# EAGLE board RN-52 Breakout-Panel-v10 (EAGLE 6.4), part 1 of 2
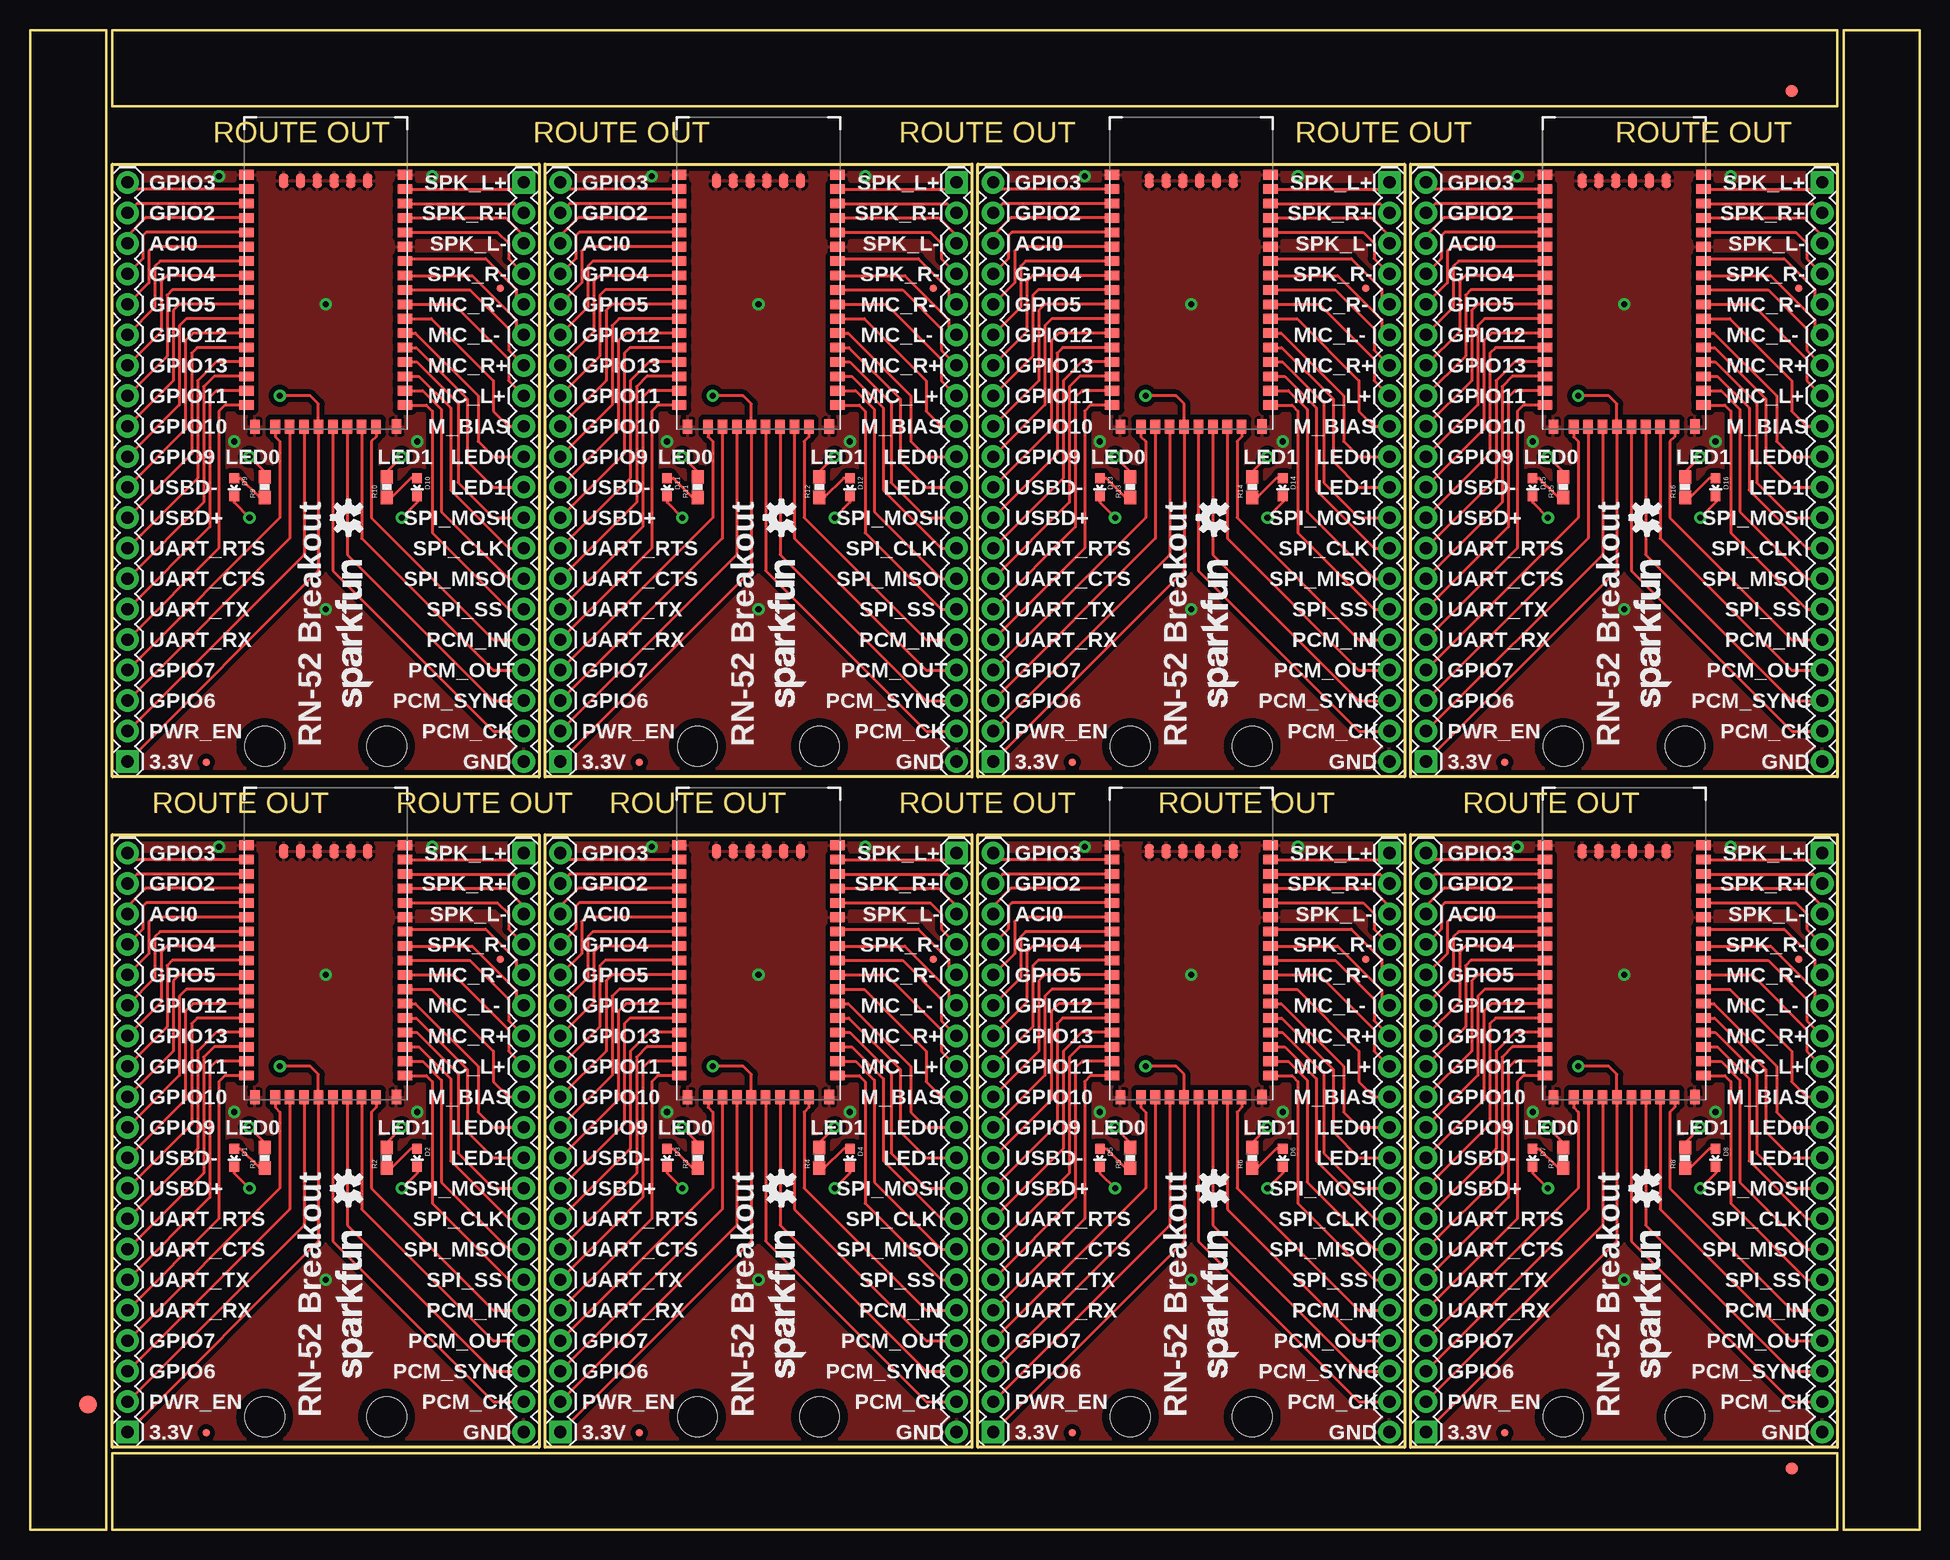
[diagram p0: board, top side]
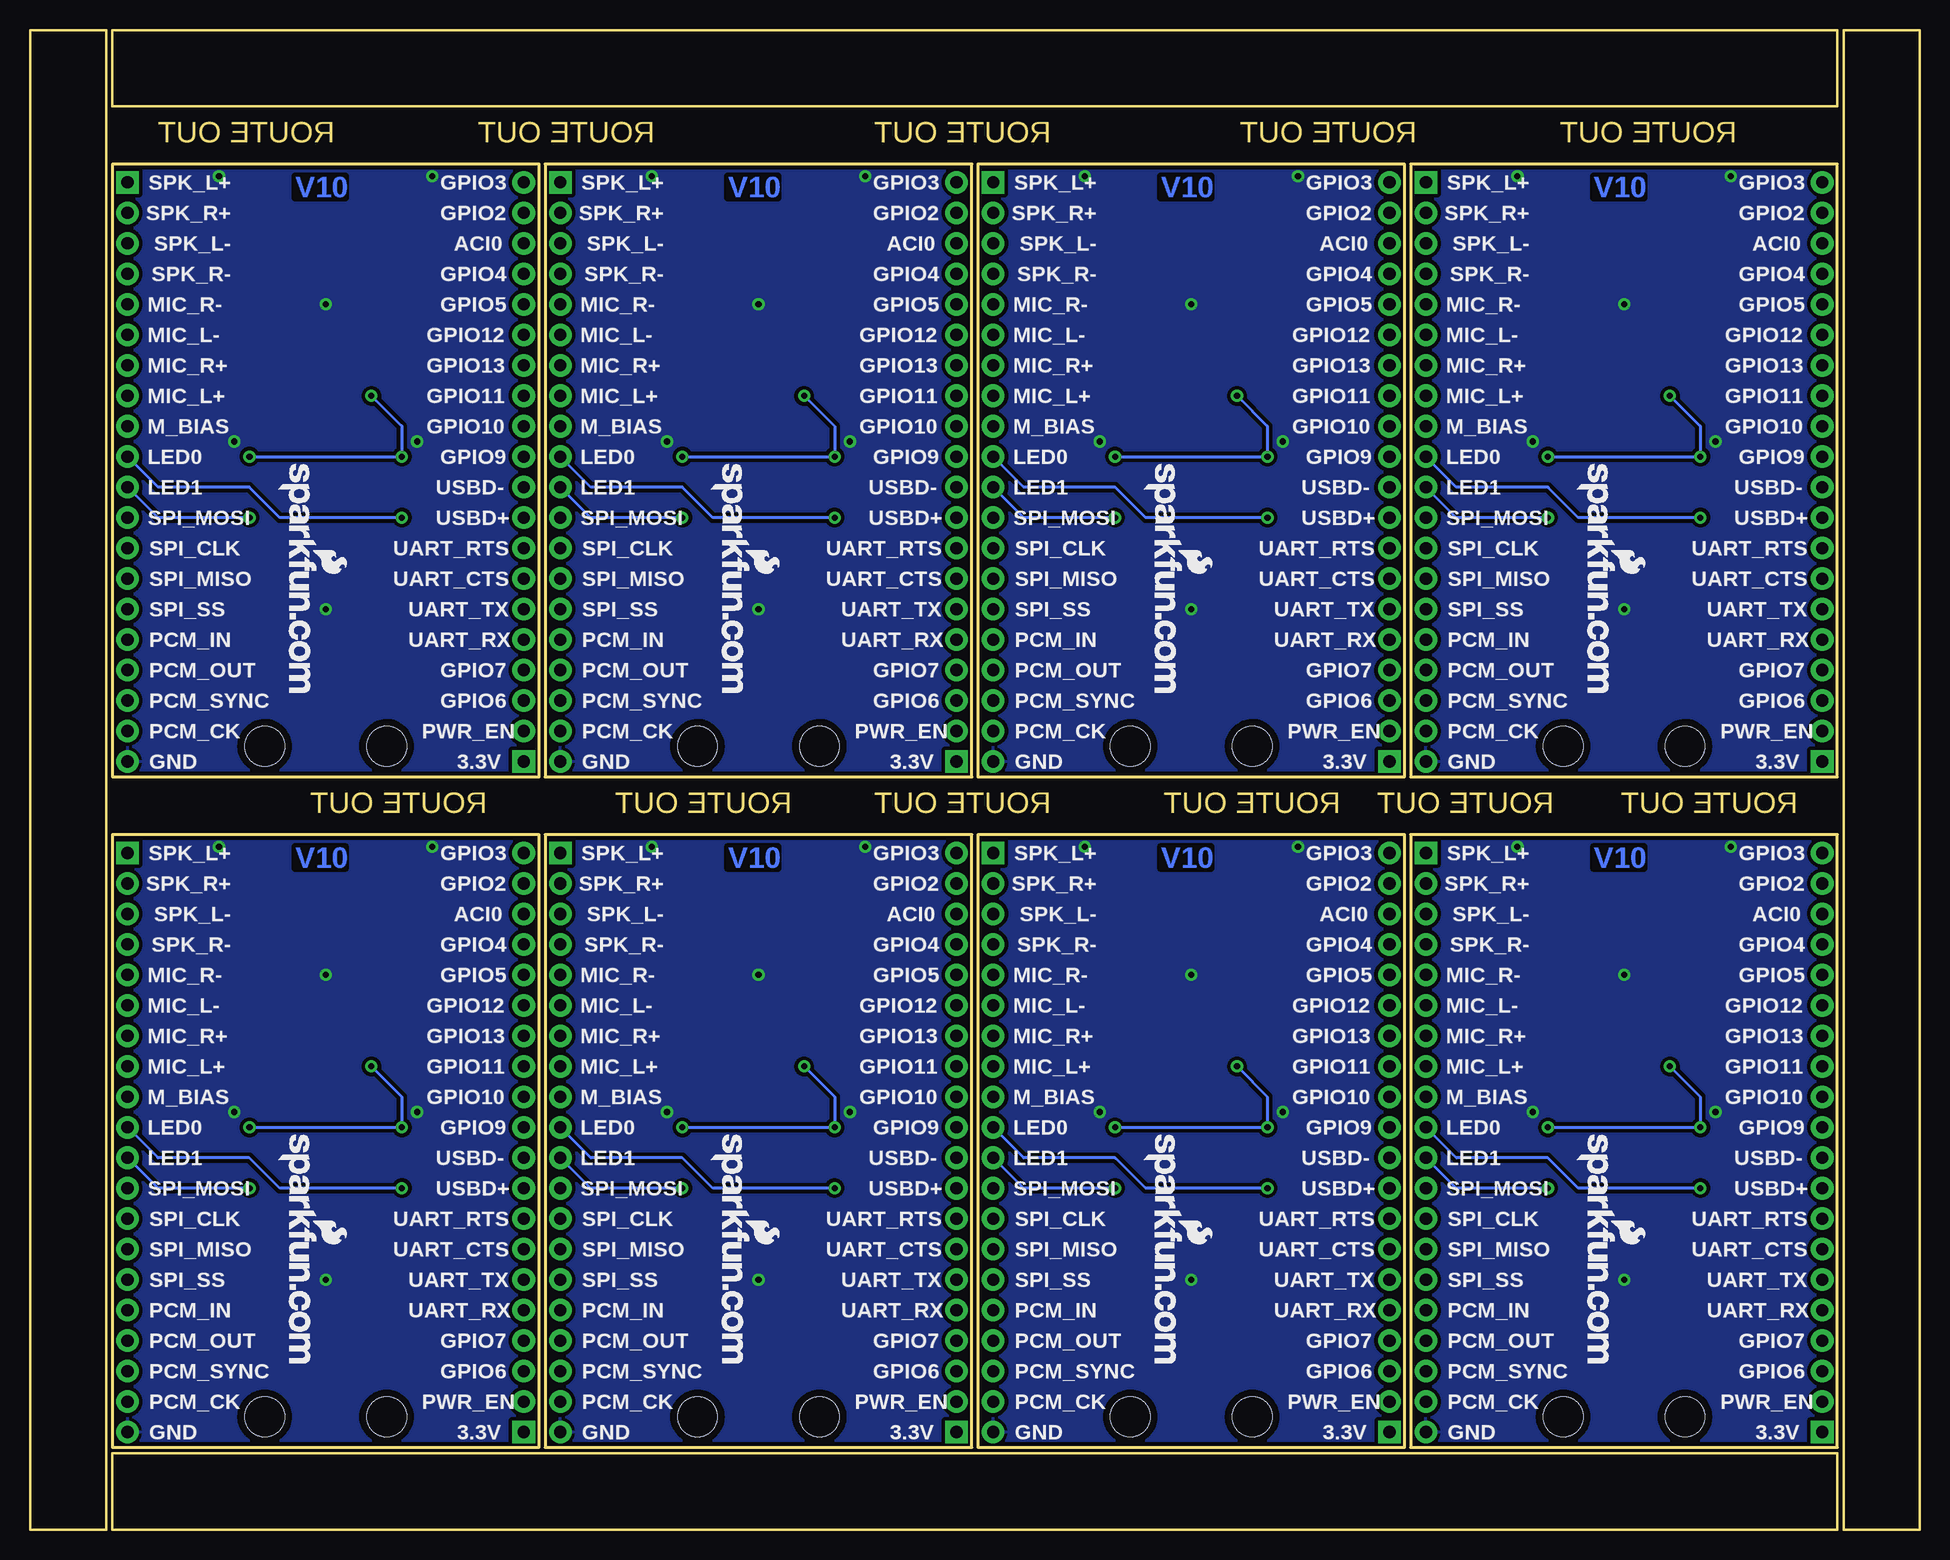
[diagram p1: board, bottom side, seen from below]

Size 157.48 x 124.97 mm. Coordinates in mm from the lower left corner, seen from the top.
Outline: 6.86,57.91 42.42,57.91 42.42,6.86 6.86,6.86 6.86,57.91
Outline: 42.93,57.91 78.49,57.91 78.49,6.86 42.93,6.86 42.93,57.91
Outline: 78.99,57.91 114.55,57.91 114.55,6.86 78.99,6.86 78.99,57.91
Outline: 115.06,57.91 150.62,57.91 150.62,6.86 115.06,6.86 115.06,57.91
Outline: 6.86,113.79 42.42,113.79 42.42,62.74 6.86,62.74 6.86,113.79
Outline: 42.93,113.79 78.49,113.79 78.49,62.74 42.93,62.74 42.93,113.79
Outline: 78.99,113.79 114.55,113.79 114.55,62.74 78.99,62.74 78.99,113.79
Outline: 115.06,113.79 150.62,113.79 150.62,62.74 115.06,62.74 115.06,113.79
Outline: 6.35,0 6.35,124.97 0,124.97 0,0 6.35,0
Outline: 6.86,0 150.62,0 150.62,6.35 6.86,6.35 6.86,0
Outline: 157.48,0 157.48,124.97 151.13,124.97 151.13,0 157.48,0
Outline: 6.86,118.62 150.62,118.62 150.62,124.97 6.86,124.97 6.86,118.62
Copper layers (1*16): Top 0.035mm / dielectric 1.5mm / Bottom 0.035mm
Design rules "default *": minimum track width 7mil, minimum drill 15mil, track to track 8mil, track to pad 8mil, pad to pad 8mil, via to via 8mil, smd to smd 8mil, copper to edge 8mil, drill to drill 8mil, minimum pad ring 12mil, minimum via ring 10mil, stop-mask expansion 4mil, vias tented up to drill 20mil, thermal gap 10mil

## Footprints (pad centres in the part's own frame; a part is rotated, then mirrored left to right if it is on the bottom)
LED-0603 = smd 0.8 x 0.8: A 0,-0.75; C 0,0.75
MICRO-FIDUCIAL = smd 0.635 x 0.635: 1 0,0
FIDUCIAL-1.5X3 = smd 1.5 x 1.5: 1 0,0
FIDUCIAL-1X2 = smd 1 x 1: 1 0,0
1X20 = drill 1.016 pad 1.88 square: 1 0,0 | drill 1.016 pad 1.88: 2 2.54,0; 3 5.08,0; 4 7.62,0; 5 10.16,0; 6 12.7,0; 7 15.24,0; 8 17.78,0; 9 20.32,0; 10 22.86,0; 11 25.4,0; 12 27.94,0; 13 30.48,0; 14 33.02,0; 15 35.56,0; 16 38.1,0; 17 40.64,0; 18 43.18,0; 19 45.72,0; 20 48.26,0
0603-RES = smd 1.1 x 1: 1 -0.85,0; 2 0.85,0
STAND-OFF = hole 3.302: 0,0
RN-52 = smd 1.2 x 0.8: 1 -6.6,8.33; 2 -6.6,7.13; 3 -6.6,5.93; 4 -6.6,4.73; 5 -6.6,3.53; 6 -6.6,2.33; 7 -6.6,1.13; 8 -6.6,-0.07; 9 -6.6,-1.27; 10 -6.6,-2.47; 11 -6.6,-3.67; 12 -6.6,-4.87; 13 -6.6,-6.07; 14 -6.6,-7.27; 15 -6.6,-8.47; 16 -6.6,-9.67; 25 6.6,-9.67; 26 6.6,-8.47; 27 6.6,-7.27; 28 6.6,-6.07; 29 6.6,-4.87; 30 6.6,-3.67; 31 6.6,-2.47; 32 6.6,-1.27; 33 6.6,-0.07; 34 6.6,1.13; 35 6.6,2.33; 36 6.6,3.53; 37 6.6,4.73; 38 6.6,5.93; 39 6.6,7.13; 40 6.6,8.33; G1 -6.6,9.53; G4 6.6,9.53 | smd 0.8 x 1.2: 17 -4.2,-11.47; 18 -3,-11.47; 19 -1.8,-11.47; 20 -0.6,-11.47; 21 0.6,-11.47; 22 1.8,-11.47; 23 3,-11.47; 24 4.2,-11.47; G2 -5.9,-11.47; G3 5.9,-11.46; RFG1 -3.5,9.03; RFG2 -2.1,9.03; RFG3 -0.7,9.03; RFG4 0.7,9.03; RFG5 2.1,9.03; RFG6 3.5,9.03

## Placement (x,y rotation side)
D1  GREEN  [LED-0603]  17.02,30.99 180 top
D2  RED  [LED-0603]  32.26,30.99 180 top
D3  GREEN  [LED-0603]  53.09,30.99 180 top
D4  RED  [LED-0603]  68.33,30.99 180 top
D5  GREEN  [LED-0603]  89.15,30.99 180 top
D6  RED  [LED-0603]  104.39,30.99 180 top
D7  GREEN  [LED-0603]  125.22,30.99 180 top
D8  RED  [LED-0603]  140.46,30.99 180 top
D9  GREEN  [LED-0603]  17.02,86.87 180 top
D10  RED  [LED-0603]  32.26,86.87 180 top
D11  GREEN  [LED-0603]  53.09,86.87 180 top
D12  RED  [LED-0603]  68.33,86.87 180 top
D13  GREEN  [LED-0603]  89.15,86.87 180 top
D14  RED  [LED-0603]  104.39,86.87 180 top
D15  GREEN  [LED-0603]  125.22,86.87 180 top
D16  RED  [LED-0603]  140.46,86.87 180 top
E$1  [MICRO-FIDUCIAL]  14.71,8.05 0 top
E$2  [MICRO-FIDUCIAL]  39.19,47.55 0 top
E$3  [MICRO-FIDUCIAL]  50.77,8.05 0 top
E$4  [MICRO-FIDUCIAL]  75.26,47.55 0 top
E$5  [MICRO-FIDUCIAL]  86.84,8.05 0 top
E$6  [MICRO-FIDUCIAL]  111.33,47.55 0 top
E$7  [MICRO-FIDUCIAL]  122.91,8.05 0 top
E$8  [MICRO-FIDUCIAL]  147.4,47.55 0 top
E$9  [MICRO-FIDUCIAL]  14.71,63.93 0 top
E$10  [MICRO-FIDUCIAL]  39.19,103.43 0 top
E$11  [MICRO-FIDUCIAL]  50.77,63.93 0 top
E$12  [MICRO-FIDUCIAL]  75.26,103.43 0 top
E$13  [MICRO-FIDUCIAL]  86.84,63.93 0 top
E$14  [MICRO-FIDUCIAL]  111.33,103.43 0 top
E$15  [MICRO-FIDUCIAL]  122.91,63.93 0 top
E$16  [MICRO-FIDUCIAL]  147.4,103.43 0 top
E$17  [FIDUCIAL-1.5X3]  4.83,10.41 0 top
E$19  [FIDUCIAL-1X2]  146.81,5.08 90 top
E$24  [FIDUCIAL-1X2]  146.81,119.89 90 top
JP1  M20  [1X20]  8.13,8.13 90 top
JP2  M20  [1X20]  41.15,56.39 270 top
JP3  M20  [1X20]  44.2,8.13 90 top
JP4  M20  [1X20]  77.22,56.39 270 top
JP5  M20  [1X20]  80.26,8.13 90 top
JP6  M20  [1X20]  113.28,56.39 270 top
JP7  M20  [1X20]  116.33,8.13 90 top
JP8  M20  [1X20]  149.35,56.39 270 top
JP9  M20  [1X20]  8.13,64.01 90 top
JP10  M20  [1X20]  41.15,112.27 270 top
JP11  M20  [1X20]  44.2,64.01 90 top
JP12  M20  [1X20]  77.22,112.27 270 top
JP13  M20  [1X20]  80.26,64.01 90 top
JP14  M20  [1X20]  113.28,112.27 270 top
JP15  M20  [1X20]  116.33,64.01 90 top
JP16  M20  [1X20]  149.35,112.27 270 top
LOGO1  OSHW-LOGOS  [OSHW-LOGO-S]  26.54,28.45 90 top
LOGO2  OSHW-LOGOS  [OSHW-LOGO-S]  62.61,28.45 90 top
LOGO3  LOGO-SFENEW  [SFE-NEW-WEBLOGO]  28.57,32.89 270 bottom
LOGO4  LOGO-SFENW2  [SFE-NEW-WEB]  28.57,12.7 90 top
LOGO5  LOGO-SFENEW  [SFE-NEW-WEBLOGO]  64.64,32.89 270 bottom
LOGO6  LOGO-SFENW2  [SFE-NEW-WEB]  64.64,12.7 90 top
LOGO7  OSHW-LOGOS  [OSHW-LOGO-S]  98.68,28.45 90 top
LOGO8  LOGO-SFENEW  [SFE-NEW-WEBLOGO]  100.71,32.89 270 bottom
LOGO9  LOGO-SFENW2  [SFE-NEW-WEB]  100.71,12.7 90 top
LOGO10  OSHW-LOGOS  [OSHW-LOGO-S]  134.75,28.45 90 top
LOGO11  LOGO-SFENEW  [SFE-NEW-WEBLOGO]  136.78,32.89 270 bottom
LOGO12  LOGO-SFENW2  [SFE-NEW-WEB]  136.78,12.7 90 top
LOGO13  OSHW-LOGOS  [OSHW-LOGO-S]  26.54,84.33 90 top
LOGO14  LOGO-SFENEW  [SFE-NEW-WEBLOGO]  28.57,88.77 270 bottom
LOGO15  LOGO-SFENW2  [SFE-NEW-WEB]  28.57,68.58 90 top
LOGO16  OSHW-LOGOS  [OSHW-LOGO-S]  62.61,84.33 90 top
LOGO17  LOGO-SFENEW  [SFE-NEW-WEBLOGO]  64.64,88.77 270 bottom
LOGO18  LOGO-SFENW2  [SFE-NEW-WEB]  64.64,68.58 90 top
LOGO19  OSHW-LOGOS  [OSHW-LOGO-S]  98.68,84.33 90 top
LOGO20  LOGO-SFENEW  [SFE-NEW-WEBLOGO]  100.71,88.77 270 bottom
LOGO21  LOGO-SFENW2  [SFE-NEW-WEB]  100.71,68.58 90 top
LOGO22  OSHW-LOGOS  [OSHW-LOGO-S]  134.75,84.33 90 top
LOGO23  LOGO-SFENEW  [SFE-NEW-WEBLOGO]  136.78,88.77 270 bottom
LOGO24  LOGO-SFENW2  [SFE-NEW-WEB]  136.78,68.58 90 top
R1  330  [0603-RES]  19.56,30.99 90 top
R2  330  [0603-RES]  29.72,30.99 90 top
R3  330  [0603-RES]  55.63,30.99 90 top
R4  330  [0603-RES]  65.79,30.99 90 top
R5  330  [0603-RES]  91.69,30.99 90 top
R6  330  [0603-RES]  101.85,30.99 90 top
R7  330  [0603-RES]  127.76,30.99 90 top
R8  330  [0603-RES]  137.92,30.99 90 top
R9  330  [0603-RES]  19.56,86.87 90 top
R10  330  [0603-RES]  29.72,86.87 90 top
R11  330  [0603-RES]  55.63,86.87 90 top
R12  330  [0603-RES]  65.79,86.87 90 top
R13  330  [0603-RES]  91.69,86.87 90 top
R14  330  [0603-RES]  101.85,86.87 90 top
R15  330  [0603-RES]  127.76,86.87 90 top
R16  330  [0603-RES]  137.92,86.87 90 top
STANDOFF1  STAND-OFF  [STAND-OFF]  19.56,9.4 0 top
STANDOFF2  STAND-OFF  [STAND-OFF]  29.72,9.4 0 top
STANDOFF3  STAND-OFF  [STAND-OFF]  55.63,9.4 0 top
STANDOFF4  STAND-OFF  [STAND-OFF]  65.79,9.4 0 top
STANDOFF5  STAND-OFF  [STAND-OFF]  91.69,9.4 0 top
STANDOFF6  STAND-OFF  [STAND-OFF]  101.85,9.4 0 top
STANDOFF7  STAND-OFF  [STAND-OFF]  127.76,9.4 0 top
STANDOFF8  STAND-OFF  [STAND-OFF]  137.92,9.4 0 top
STANDOFF9  STAND-OFF  [STAND-OFF]  19.56,65.28 0 top
STANDOFF10  STAND-OFF  [STAND-OFF]  29.72,65.28 0 top
STANDOFF11  STAND-OFF  [STAND-OFF]  55.63,65.28 0 top
STANDOFF12  STAND-OFF  [STAND-OFF]  65.79,65.28 0 top
STANDOFF13  STAND-OFF  [STAND-OFF]  91.69,65.28 0 top
STANDOFF14  STAND-OFF  [STAND-OFF]  101.85,65.28 0 top
STANDOFF15  STAND-OFF  [STAND-OFF]  127.76,65.28 0 top
STANDOFF16  STAND-OFF  [STAND-OFF]  137.92,65.28 0 top
U1  BLUETOOTH-RN-52  [RN-52]  24.64,47.5 0 top
U2  BLUETOOTH-RN-52  [RN-52]  60.71,47.5 0 top
U3  BLUETOOTH-RN-52  [RN-52]  96.77,47.5 0 top
U4  BLUETOOTH-RN-52  [RN-52]  132.84,47.5 0 top
U5  BLUETOOTH-RN-52  [RN-52]  24.64,103.38 0 top
U6  BLUETOOTH-RN-52  [RN-52]  60.71,103.38 0 top
U7  BLUETOOTH-RN-52  [RN-52]  96.77,103.38 0 top
U8  BLUETOOTH-RN-52  [RN-52]  132.84,103.38 0 top

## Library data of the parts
D1 D3 D5 D7 D9 D11 D13 D15 = SparkFun-LED; PROD_ID: DIO-00821
D2 D4 D6 D8 D10 D12 D14 D16 = SparkFun-LED; PROD_ID: DIO-00819
E$1-E$17 E$19 E$24 LOGO1-LOGO24 = SparkFun-Aesthetics
JP1-JP16 = SparkFun-Connectors
R1-R16 = SparkFun-Resistors
STANDOFF1-STANDOFF16 = SparkFun-Electromechanical
U1-U8 = SparkFun-RF

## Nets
3.3V: JP1.1 R1.2 R2.2 U1.20
3.3V1: JP3.1 R3.2 R4.2 U2.20
3.3V2: JP5.1 R5.2 R6.2 U3.20
3.3V3: JP7.1 R7.2 R8.2 U4.20
3.3V4: JP9.1 R9.2 R10.2 U5.20
3.3V5: JP11.1 R11.2 R12.2 U6.20
3.3V6: JP13.1 R13.2 R14.2 U7.20
3.3V7: JP15.1 R15.2 R16.2 U8.20
AIC0: JP1.18 U1.3
AIC1: JP3.18 U2.3
AIC2: JP5.18 U3.3
AIC3: JP7.18 U4.3
AIC4: JP9.18 U5.3
AIC5: JP11.18 U6.3
AIC6: JP13.18 U7.3
AIC7: JP15.18 U8.3
GND: JP2.20 U1.36 U1.G1 U1.G2 U1.G3 U1.G4 U1.RFG1 U1.RFG2 U1.RFG3 U1.RFG4 U1.RFG5 U1.RFG6
GND1: JP4.20 U2.36 U2.G1 U2.G2 U2.G3 U2.G4 U2.RFG1 U2.RFG2 U2.RFG3 U2.RFG4 U2.RFG5 U2.RFG6
GND2: JP6.20 U3.36 U3.G1 U3.G2 U3.G3 U3.G4 U3.RFG1 U3.RFG2 U3.RFG3 U3.RFG4 U3.RFG5 U3.RFG6
GND3: JP8.20 U4.36 U4.G1 U4.G2 U4.G3 U4.G4 U4.RFG1 U4.RFG2 U4.RFG3 U4.RFG4 U4.RFG5 U4.RFG6
GND4: JP10.20 U5.36 U5.G1 U5.G2 U5.G3 U5.G4 U5.RFG1 U5.RFG2 U5.RFG3 U5.RFG4 U5.RFG5 U5.RFG6
GND5: JP12.20 U6.36 U6.G1 U6.G2 U6.G3 U6.G4 U6.RFG1 U6.RFG2 U6.RFG3 U6.RFG4 U6.RFG5 U6.RFG6
GND6: JP14.20 U7.36 U7.G1 U7.G2 U7.G3 U7.G4 U7.RFG1 U7.RFG2 U7.RFG3 U7.RFG4 U7.RFG5 U7.RFG6
GND7: JP16.20 U8.36 U8.G1 U8.G2 U8.G3 U8.G4 U8.RFG1 U8.RFG2 U8.RFG3 U8.RFG4 U8.RFG5 U8.RFG6
GPIO1: JP3.20 U2.1
GPIO2: JP1.19 U1.2
GPIO3: JP1.20 U1.1
GPIO4: JP1.17 U1.4
GPIO5: JP1.16 U1.5
GPIO6: JP1.3 U1.18
GPIO7: JP1.4 U1.17
GPIO8: JP3.19 U2.2
GPIO9: JP1.11 U1.10
GPIO10: JP1.12 U1.9
GPIO11: JP1.13 U1.8
GPIO12: JP1.15 U1.6
GPIO13: JP1.14 U1.7
GPIO14: JP3.17 U2.4
GPIO15: JP3.16 U2.5
GPIO16: JP3.15 U2.6
GPIO17: JP3.14 U2.7
GPIO18: JP3.13 U2.8
GPIO19: JP3.12 U2.9
GPIO20: JP3.11 U2.10
GPIO21: JP3.4 U2.17
GPIO22: JP3.3 U2.18
GPIO23: JP5.20 U3.1
GPIO24: JP5.19 U3.2
GPIO25: JP5.17 U3.4
GPIO26: JP5.16 U3.5
GPIO27: JP5.15 U3.6
GPIO28: JP5.14 U3.7
GPIO29: JP5.13 U3.8
GPIO30: JP5.12 U3.9
GPIO31: JP5.11 U3.10
GPIO32: JP5.4 U3.17
GPIO33: JP5.3 U3.18
GPIO34: JP7.20 U4.1
GPIO35: JP7.19 U4.2
GPIO36: JP7.17 U4.4
GPIO37: JP7.16 U4.5
GPIO38: JP7.15 U4.6
GPIO39: JP7.14 U4.7
GPIO40: JP7.13 U4.8
GPIO41: JP7.12 U4.9
GPIO42: JP7.11 U4.10
GPIO43: JP7.4 U4.17
GPIO44: JP7.3 U4.18
GPIO45: JP9.20 U5.1
GPIO46: JP9.19 U5.2
GPIO47: JP9.17 U5.4
GPIO48: JP9.16 U5.5
GPIO49: JP9.15 U5.6
GPIO50: JP9.14 U5.7
GPIO51: JP9.13 U5.8
GPIO52: JP9.12 U5.9
GPIO53: JP9.11 U5.10
GPIO54: JP9.4 U5.17
GPIO55: JP9.3 U5.18
GPIO56: JP11.20 U6.1
GPIO57: JP11.19 U6.2
GPIO58: JP11.17 U6.4
GPIO59: JP11.16 U6.5
GPIO60: JP11.15 U6.6
GPIO61: JP11.14 U6.7
GPIO62: JP11.13 U6.8
GPIO63: JP11.12 U6.9
GPIO64: JP11.11 U6.10
GPIO65: JP11.4 U6.17
GPIO66: JP11.3 U6.18
GPIO67: JP13.20 U7.1
GPIO68: JP13.19 U7.2
GPIO69: JP13.17 U7.4
GPIO70: JP13.16 U7.5
GPIO71: JP13.15 U7.6
GPIO72: JP13.14 U7.7
GPIO73: JP13.13 U7.8
GPIO74: JP13.12 U7.9
GPIO75: JP13.11 U7.10
GPIO76: JP13.4 U7.17
GPIO77: JP13.3 U7.18
GPIO78: JP15.20 U8.1
GPIO79: JP15.19 U8.2
GPIO80: JP15.17 U8.4
GPIO81: JP15.16 U8.5
GPIO82: JP15.15 U8.6
GPIO83: JP15.14 U8.7
GPIO84: JP15.13 U8.8
GPIO85: JP15.12 U8.9
GPIO86: JP15.11 U8.10
GPIO87: JP15.4 U8.17
GPIO88: JP15.3 U8.18
LED0: D1.C JP2.10 U1.30
LED1: D2.C JP2.11 U1.29
LED2: D3.C JP4.10 U2.30
LED3: D4.C JP4.11 U2.29
LED4: D5.C JP6.10 U3.30
LED5: D6.C JP6.11 U3.29
LED6: D7.C JP8.10 U4.30
LED7: D8.C JP8.11 U4.29
LED8: D9.C JP10.10 U5.30
LED9: D10.C JP10.11 U5.29
LED10: D11.C JP12.10 U6.30
LED11: D12.C JP12.11 U6.29
LED12: D13.C JP14.10 U7.30
LED13: D14.C JP14.11 U7.29
LED14: D15.C JP16.10 U8.30
LED15: D16.C JP16.11 U8.29
MIC_BIAS: JP2.9 U1.31
MIC_BIAS1: JP4.9 U2.31
MIC_BIAS2: JP6.9 U3.31
MIC_BIAS3: JP8.9 U4.31
MIC_BIAS4: JP10.9 U5.31
MIC_BIAS5: JP12.9 U6.31
MIC_BIAS6: JP14.9 U7.31
MIC_BIAS7: JP16.9 U8.31
MIC_L+: JP2.8 U1.32
MIC_L+1: JP4.8 U2.32
MIC_L+2: JP6.8 U3.32
MIC_L+3: JP8.8 U4.32
MIC_L+4: JP10.8 U5.32
MIC_L+5: JP12.8 U6.32
MIC_L+6: JP14.8 U7.32
MIC_L+7: JP16.8 U8.32
MIC_L-: JP2.6 U1.34
MIC_L-1: JP4.6 U2.34
MIC_L-2: JP6.6 U3.34
MIC_L-3: JP8.6 U4.34
MIC_L-4: JP10.6 U5.34
MIC_L-5: JP12.6 U6.34
MIC_L-6: JP14.6 U7.34
MIC_L-7: JP16.6 U8.34
MIC_R+: JP2.7 U1.33
MIC_R+1: JP4.7 U2.33
MIC_R+2: JP6.7 U3.33
MIC_R+3: JP8.7 U4.33
MIC_R+4: JP10.7 U5.33
MIC_R+5: JP12.7 U6.33
MIC_R+6: JP14.7 U7.33
MIC_R+7: JP16.7 U8.33
MIC_R-: JP2.5 U1.35
MIC_R-1: JP4.5 U2.35
MIC_R-2: JP6.5 U3.35
MIC_R-3: JP8.5 U4.35
MIC_R-4: JP10.5 U5.35
MIC_R-5: JP12.5 U6.35
MIC_R-6: JP14.5 U7.35
MIC_R-7: JP16.5 U8.35
N$1: D2.A R2.1
N$2: D1.A R1.1
N$3: D4.A R4.1
N$4: D3.A R3.1
N$5: D6.A R6.1
N$6: D5.A R5.1
N$7: D8.A R8.1
N$8: D7.A R7.1
N$9: D10.A R10.1
N$10: D9.A R9.1
N$11: D12.A R12.1
N$12: D11.A R11.1
N$13: D14.A R14.1
N$14: D13.A R13.1
N$15: D16.A R16.1
N$16: D15.A R15.1
PCM_CLK: JP2.16 U1.24
PCM_CLK1: JP4.16 U2.24
PCM_CLK2: JP6.16 U3.24
PCM_CLK3: JP8.16 U4.24
PCM_CLK4: JP10.16 U5.24
PCM_CLK5: JP12.16 U6.24
PCM_CLK6: JP14.16 U7.24
PCM_CLK7: JP16.16 U8.24
PCM_IN: JP2.19 U1.21
PCM_IN1: JP4.19 U2.21
PCM_IN2: JP6.19 U3.21
PCM_IN3: JP8.19 U4.21
PCM_IN4: JP10.19 U5.21
PCM_IN5: JP12.19 U6.21
PCM_IN6: JP14.19 U7.21
PCM_IN7: JP16.19 U8.21
PCM_OUT: JP2.18 U1.22
PCM_OUT1: JP4.18 U2.22
PCM_OUT2: JP6.18 U3.22
PCM_OUT3: JP8.18 U4.22
PCM_OUT4: JP10.18 U5.22
PCM_OUT5: JP12.18 U6.22
PCM_OUT6: JP14.18 U7.22
PCM_OUT7: JP16.18 U8.22
PCM_SYNC: JP2.17 U1.23
PCM_SYNC1: JP4.17 U2.23
PCM_SYNC2: JP6.17 U3.23
PCM_SYNC3: JP8.17 U4.23
PCM_SYNC4: JP10.17 U5.23
PCM_SYNC5: JP12.17 U6.23
PCM_SYNC6: JP14.17 U7.23
PCM_SYNC7: JP16.17 U8.23
PWREN: JP1.2 U1.19
PWREN1: JP3.2 U2.19
PWREN2: JP5.2 U3.19
PWREN3: JP7.2 U4.19
PWREN4: JP9.2 U5.19
PWREN5: JP11.2 U6.19
PWREN6: JP13.2 U7.19
PWREN7: JP15.2 U8.19
SPI_CLK: JP2.13 U1.27
SPI_CLK1: JP4.13 U2.27
SPI_CLK2: JP6.13 U3.27
SPI_CLK3: JP8.13 U4.27
SPI_CLK4: JP10.13 U5.27
SPI_CLK5: JP12.13 U6.27
SPI_CLK6: JP14.13 U7.27
SPI_CLK7: JP16.13 U8.27
SPI_MISO: JP2.14 U1.26
SPI_MISO1: JP4.14 U2.26
SPI_MISO2: JP6.14 U3.26
SPI_MISO3: JP8.14 U4.26
SPI_MISO4: JP10.14 U5.26
SPI_MISO5: JP12.14 U6.26
SPI_MISO6: JP14.14 U7.26
SPI_MISO7: JP16.14 U8.26
SPI_MOSI: JP2.12 U1.28
SPI_MOSI1: JP4.12 U2.28
SPI_MOSI2: JP6.12 U3.28
SPI_MOSI3: JP8.12 U4.28
SPI_MOSI4: JP10.12 U5.28
SPI_MOSI5: JP12.12 U6.28
SPI_MOSI6: JP14.12 U7.28
SPI_MOSI7: JP16.12 U8.28
SPI_SS: JP2.15 U1.25
SPI_SS1: JP4.15 U2.25
SPI_SS2: JP6.15 U3.25
SPI_SS3: JP8.15 U4.25
SPI_SS4: JP10.15 U5.25
SPI_SS5: JP12.15 U6.25
SPI_SS6: JP14.15 U7.25
SPI_SS7: JP16.15 U8.25
SPKR_L+: JP2.1 U1.40
SPKR_L+1: JP4.1 U2.40
SPKR_L+2: JP6.1 U3.40
SPKR_L+3: JP8.1 U4.40
SPKR_L+4: JP10.1 U5.40
SPKR_L+5: JP12.1 U6.40
SPKR_L+6: JP14.1 U7.40
SPKR_L+7: JP16.1 U8.40
SPKR_L-: JP2.3 U1.38
SPKR_L-1: JP4.3 U2.38
SPKR_L-2: JP6.3 U3.38
SPKR_L-3: JP8.3 U4.38
SPKR_L-4: JP10.3 U5.38
SPKR_L-5: JP12.3 U6.38
SPKR_L-6: JP14.3 U7.38
SPKR_L-7: JP16.3 U8.38
SPKR_R+: JP2.2 U1.39
SPKR_R+1: JP4.2 U2.39
SPKR_R+2: JP6.2 U3.39
SPKR_R+3: JP8.2 U4.39
SPKR_R+4: JP10.2 U5.39
SPKR_R+5: JP12.2 U6.39
SPKR_R+6: JP14.2 U7.39
SPKR_R+7: JP16.2 U8.39
SPKR_R-: JP2.4 U1.37
SPKR_R-1: JP4.4 U2.37
SPKR_R-2: JP6.4 U3.37
SPKR_R-3: JP8.4 U4.37
SPKR_R-4: JP10.4 U5.37
SPKR_R-5: JP12.4 U6.37
SPKR_R-6: JP14.4 U7.37
SPKR_R-7: JP16.4 U8.37
UART_CTS: JP1.7 U1.14
UART_CTS1: JP3.7 U2.14
UART_CTS2: JP5.7 U3.14
UART_CTS3: JP7.7 U4.14
UART_CTS4: JP9.7 U5.14
UART_CTS5: JP11.7 U6.14
UART_CTS6: JP13.7 U7.14
UART_CTS7: JP15.7 U8.14
UART_RTS: JP1.8 U1.13
UART_RTS1: JP3.8 U2.13
UART_RTS2: JP5.8 U3.13
UART_RTS3: JP7.8 U4.13
UART_RTS4: JP9.8 U5.13
UART_RTS5: JP11.8 U6.13
UART_RTS6: JP13.8 U7.13
UART_RTS7: JP15.8 U8.13
UART_RX: JP1.5 U1.16
UART_RX1: JP3.5 U2.16
UART_RX2: JP5.5 U3.16
UART_RX3: JP7.5 U4.16
UART_RX4: JP9.5 U5.16
UART_RX5: JP11.5 U6.16
UART_RX6: JP13.5 U7.16
UART_RX7: JP15.5 U8.16
UART_TX: JP1.6 U1.15
UART_TX1: JP3.6 U2.15
UART_TX2: JP5.6 U3.15
UART_TX3: JP7.6 U4.15
UART_TX4: JP9.6 U5.15
UART_TX5: JP11.6 U6.15
UART_TX6: JP13.6 U7.15
UART_TX7: JP15.6 U8.15
USBD+: JP1.9 U1.12
USBD+1: JP3.9 U2.12
USBD+2: JP5.9 U3.12
USBD+3: JP7.9 U4.12
USBD+4: JP9.9 U5.12
USBD+5: JP11.9 U6.12
USBD+6: JP13.9 U7.12
USBD+7: JP15.9 U8.12
USBD-: JP1.10 U1.11
USBD-1: JP3.10 U2.11
USBD-2: JP5.10 U3.11
USBD-3: JP7.10 U4.11
USBD-4: JP9.10 U5.11
USBD-5: JP11.10 U6.11
USBD-6: JP13.10 U7.11
USBD-7: JP15.10 U8.11

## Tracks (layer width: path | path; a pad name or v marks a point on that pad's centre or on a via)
3.3V  (via drill 0.51)
  Top 0.254: JP1.1 24.04,24.04 U1.20 24.04,37.94 23.37,38.61 v20.83,38.61 | R2.2 29.72,32.26 v30.99,33.53 | R1.2 19.56,32.26 v18.29,33.53
  Bottom 0.254: v30.99,33.53 v18.29,33.53 18.29,36.07 v20.83,38.61
3.3V1  (via drill 0.51)
  Top 0.254: JP3.1 60.11,24.04 U2.20 60.11,37.94 59.44,38.61 v56.9,38.61 | R4.2 65.79,32.26 v67.06,33.53 | R3.2 55.63,32.26 v54.36,33.53
  Bottom 0.254: v67.06,33.53 v54.36,33.53 54.36,36.07 v56.9,38.61
3.3V2  (via drill 0.51)
  Top 0.254: JP5.1 96.17,24.04 U3.20 96.17,37.94 95.5,38.61 v92.96,38.61 | R6.2 101.85,32.26 v103.12,33.53 | R5.2 91.69,32.26 v90.42,33.53
  Bottom 0.254: v103.12,33.53 v90.42,33.53 90.42,36.07 v92.96,38.61
3.3V3  (via drill 0.51)
  Top 0.254: JP7.1 132.24,24.04 U4.20 132.24,37.94 131.57,38.61 v129.03,38.61 | R8.2 137.92,32.26 v139.19,33.53 | R7.2 127.76,32.26 v126.49,33.53
  Bottom 0.254: v139.19,33.53 v126.49,33.53 126.49,36.07 v129.03,38.61
3.3V4  (via drill 0.51)
  Top 0.254: JP9.1 24.04,79.92 U5.20 24.04,93.82 23.37,94.49 v20.83,94.49 | R10.2 29.72,88.14 v30.99,89.41 | R9.2 19.56,88.14 v18.29,89.41
  Bottom 0.254: v30.99,89.41 v18.29,89.41 18.29,91.95 v20.83,94.49
3.3V5  (via drill 0.51)
  Top 0.254: JP11.1 60.11,79.92 U6.20 60.11,93.82 59.44,94.49 v56.9,94.49 | R12.2 65.79,88.14 v67.06,89.41 | R11.2 55.63,88.14 v54.36,89.41
  Bottom 0.254: v67.06,89.41 v54.36,89.41 54.36,91.95 v56.9,94.49
3.3V6  (via drill 0.51)
  Top 0.254: JP13.1 96.17,79.92 U7.20 96.17,93.82 95.5,94.49 v92.96,94.49 | R14.2 101.85,88.14 v103.12,89.41 | R13.2 91.69,88.14 v90.42,89.41
  Bottom 0.254: v103.12,89.41 v90.42,89.41 90.42,91.95 v92.96,94.49
3.3V7  (via drill 0.51)
  Top 0.254: JP15.1 132.24,79.92 U8.20 132.24,93.82 131.57,94.49 v129.03,94.49 | R16.2 137.92,88.14 v139.19,89.41 | R15.2 127.76,88.14 v126.49,89.41
  Bottom 0.254: v139.19,89.41 v126.49,89.41 126.49,91.95 v129.03,94.49
AIC0
  Top 0.254: U1.3 9.61,53.43 8.13,51.94 JP1.18
AIC1
  Top 0.254: U2.3 45.68,53.43 44.2,51.94 JP3.18
AIC2
  Top 0.254: U3.3 81.75,53.43 80.26,51.94 JP5.18
AIC3
  Top 0.254: U4.3 117.82,53.43 116.33,51.94 JP7.18
AIC4
  Top 0.254: U5.3 9.61,109.31 8.13,107.82 JP9.18
AIC5
  Top 0.254: U6.3 45.68,109.31 44.2,107.82 JP11.18
AIC6
  Top 0.254: U7.3 81.75,109.31 80.26,107.82 JP13.18
AIC7
  Top 0.254: U8.3 117.82,109.31 116.33,107.82 JP15.18
GND  (via drill 0.51)
  other vias: 24.64,46.23 24.64,20.83 17.02,34.8 32.26,34.8 33.53,56.9 15.75,56.9
  pour Bottom (isolate 0.305): 6.86,57.66 42.42,57.66 42.42,6.86 6.86,6.86
  pour Top (isolate 0.406): 6.86,57.66 42.42,57.66 42.42,6.86 6.86,6.86
GND1  (via drill 0.51)
  other vias: 60.71,46.23 60.71,20.83 53.09,34.8 68.33,34.8 69.6,56.9 51.82,56.9
  pour Bottom (isolate 0.305): 42.93,57.66 78.49,57.66 78.49,6.86 42.93,6.86
  pour Top (isolate 0.406): 42.93,57.66 78.49,57.66 78.49,6.86 42.93,6.86
GND2  (via drill 0.51)
  other vias: 96.77,46.23 96.77,20.83 89.15,34.8 104.39,34.8 105.66,56.9 87.88,56.9
  pour Bottom (isolate 0.305): 78.99,57.66 114.55,57.66 114.55,6.86 78.99,6.86
  pour Top (isolate 0.406): 78.99,57.66 114.55,57.66 114.55,6.86 78.99,6.86
GND3  (via drill 0.51)
  other vias: 132.84,46.23 132.84,20.83 125.22,34.8 140.46,34.8 141.73,56.9 123.95,56.9
  pour Bottom (isolate 0.305): 115.06,57.66 150.62,57.66 150.62,6.86 115.06,6.86
  pour Top (isolate 0.406): 115.06,57.66 150.62,57.66 150.62,6.86 115.06,6.86
GND4  (via drill 0.51)
  other vias: 24.64,102.11 24.64,76.71 17.02,90.68 32.26,90.68 33.53,112.78 15.75,112.78
  pour Bottom (isolate 0.305): 6.86,113.54 42.42,113.54 42.42,62.74 6.86,62.74
  pour Top (isolate 0.406): 6.86,113.54 42.42,113.54 42.42,62.74 6.86,62.74
GND5  (via drill 0.51)
  other vias: 60.71,102.11 60.71,76.71 53.09,90.68 68.33,90.68 69.6,112.78 51.82,112.78
  pour Bottom (isolate 0.305): 42.93,113.54 78.49,113.54 78.49,62.74 42.93,62.74
  pour Top (isolate 0.406): 42.93,113.54 78.49,113.54 78.49,62.74 42.93,62.74
GND6  (via drill 0.51)
  other vias: 96.77,102.11 96.77,76.71 89.15,90.68 104.39,90.68 105.66,112.78 87.88,112.78
  pour Bottom (isolate 0.305): 78.99,113.54 114.55,113.54 114.55,62.74 78.99,62.74
  pour Top (isolate 0.406): 78.99,113.54 114.55,113.54 114.55,62.74 78.99,62.74
GND7  (via drill 0.51)
  other vias: 132.84,102.11 132.84,76.71 125.22,90.68 140.46,90.68 141.73,112.78 123.95,112.78
  pour Bottom (isolate 0.305): 115.06,113.54 150.62,113.54 150.62,62.74 115.06,62.74
  pour Top (isolate 0.406): 115.06,113.54 150.62,113.54 150.62,62.74 115.06,62.74
GPIO1
  Top 0.254: U2.1 44.76,55.83 JP3.20
GPIO2
  Top 0.254: U1.2 8.91,54.63 JP1.19
GPIO3
  Top 0.254: U1.1 8.69,55.83 JP1.20
GPIO4
  Top 0.254: U1.4 9.68,52.23 9.4,51.94 9.4,50.04 JP1.17
GPIO5
  Top 0.254: U1.5 10.26,51.03 9.91,50.67 9.91,48.01 JP1.16
GPIO6
  Top 0.254: U1.18 21.64,26.72 JP1.3
GPIO7
  Top 0.254: U1.17 20.44,35.19 20.83,34.8 20.83,28.45 JP1.4
GPIO8
  Top 0.254: U2.2 44.98,54.63 JP3.19
GPIO9
  Top 0.254: U1.10 13.02,45.03 12.45,44.45 12.45,37.85 JP1.11
GPIO10
  Top 0.254: U1.9 12.45,46.23 11.94,45.72 11.94,39.88 JP1.12
GPIO11
  Top 0.254: U1.8 11.87,47.43 11.43,46.99 11.43,41.91 JP1.13
GPIO12
  Top 0.254: U1.6 10.84,49.83 10.41,49.4 10.41,45.97 JP1.15
GPIO13
  Top 0.254: U1.7 11.42,48.63 10.92,48.13 10.92,43.94 JP1.14
GPIO14
  Top 0.254: U2.4 45.75,52.23 45.47,51.94 45.47,50.04 JP3.17
GPIO15
  Top 0.254: U2.5 46.33,51.03 45.97,50.67 45.97,48.01 JP3.16
GPIO16
  Top 0.254: U2.6 46.91,49.83 46.48,49.4 46.48,45.97 JP3.15
GPIO17
  Top 0.254: U2.7 47.48,48.63 46.99,48.13 46.99,43.94 JP3.14
GPIO18
  Top 0.254: U2.8 47.94,47.43 47.5,46.99 47.5,41.91 JP3.13
GPIO19
  Top 0.254: U2.9 48.51,46.23 48.01,45.72 48.01,39.88 JP3.12
GPIO20
  Top 0.254: U2.10 49.09,45.03 48.51,44.45 48.51,37.85 JP3.11
GPIO21
  Top 0.254: U2.17 56.51,35.19 56.9,34.8 56.9,28.45 JP3.4
GPIO22
  Top 0.254: U2.18 57.71,26.72 JP3.3
GPIO23
  Top 0.254: U3.1 80.82,55.83 JP5.20
GPIO24
  Top 0.254: U3.2 81.04,54.63 JP5.19
GPIO25
  Top 0.254: U3.4 81.82,52.23 81.53,51.94 81.53,50.04 JP5.17
GPIO26
  Top 0.254: U3.5 82.4,51.03 82.04,50.67 82.04,48.01 JP5.16
GPIO27
  Top 0.254: U3.6 82.97,49.83 82.55,49.4 82.55,45.97 JP5.15
GPIO28
  Top 0.254: U3.7 83.55,48.63 83.06,48.13 83.06,43.94 JP5.14
GPIO29
  Top 0.254: U3.8 84,47.43 83.57,46.99 83.57,41.91 JP5.13
GPIO30
  Top 0.254: U3.9 84.58,46.23 84.07,45.72 84.07,39.88 JP5.12
GPIO31
  Top 0.254: U3.10 85.16,45.03 84.58,44.45 84.58,37.85 JP5.11
GPIO32
  Top 0.254: U3.17 92.57,35.19 92.96,34.8 92.96,28.45 JP5.4
GPIO33
  Top 0.254: U3.18 93.77,26.72 JP5.3
GPIO34
  Top 0.254: U4.1 116.89,55.83 JP7.20
GPIO35
  Top 0.254: U4.2 117.11,54.63 JP7.19
GPIO36
  Top 0.254: U4.4 117.89,52.23 117.6,51.94 117.6,50.04 JP7.17
GPIO37
  Top 0.254: U4.5 118.47,51.03 118.11,50.67 118.11,48.01 JP7.16
GPIO38
  Top 0.254: U4.6 119.04,49.83 118.62,49.4 118.62,45.97 JP7.15
GPIO39
  Top 0.254: U4.7 119.62,48.63 119.13,48.13 119.13,43.94 JP7.14
GPIO40
  Top 0.254: U4.8 120.07,47.43 119.63,46.99 119.63,41.91 JP7.13
GPIO41
  Top 0.254: U4.9 120.65,46.23 120.14,45.72 120.14,39.88 JP7.12
GPIO42
  Top 0.254: U4.10 121.23,45.03 120.65,44.45 120.65,37.85 JP7.11
GPIO43
  Top 0.254: U4.17 128.64,35.19 129.03,34.8 129.03,28.45 JP7.4
GPIO44
  Top 0.254: U4.18 129.84,26.72 JP7.3
GPIO45
  Top 0.254: U5.1 8.69,111.71 JP9.20
GPIO46
  Top 0.254: U5.2 8.91,110.51 JP9.19
GPIO47
  Top 0.254: U5.4 9.68,108.11 9.4,107.82 9.4,105.92 JP9.17
GPIO48
  Top 0.254: U5.5 10.26,106.91 9.91,106.55 9.91,103.89 JP9.16
GPIO49
  Top 0.254: U5.6 10.84,105.71 10.41,105.28 10.41,101.85 JP9.15
GPIO50
  Top 0.254: U5.7 11.42,104.51 10.92,104.01 10.92,99.82 JP9.14
GPIO51
  Top 0.254: U5.8 11.87,103.31 11.43,102.87 11.43,97.79 JP9.13
GPIO52
  Top 0.254: U5.9 12.45,102.11 11.94,101.6 11.94,95.76 JP9.12
GPIO53
  Top 0.254: U5.10 13.02,100.91 12.45,100.33 12.45,93.73 JP9.11
GPIO54
  Top 0.254: U5.17 20.44,91.07 20.83,90.68 20.83,84.33 JP9.4
GPIO55
  Top 0.254: U5.18 21.64,82.6 JP9.3
GPIO56
  Top 0.254: U6.1 44.76,111.71 JP11.20
GPIO57
  Top 0.254: U6.2 44.98,110.51 JP11.19
GPIO58
  Top 0.254: U6.4 45.75,108.11 45.47,107.82 45.47,105.92 JP11.17
GPIO59
  Top 0.254: U6.5 46.33,106.91 45.97,106.55 45.97,103.89 JP11.16
GPIO60
  Top 0.254: U6.6 46.91,105.71 46.48,105.28 46.48,101.85 JP11.15
GPIO61
  Top 0.254: U6.7 47.48,104.51 46.99,104.01 46.99,99.82 JP11.14
GPIO62
  Top 0.254: U6.8 47.94,103.31 47.5,102.87 47.5,97.79 JP11.13
GPIO63
  Top 0.254: U6.9 48.51,102.11 48.01,101.6 48.01,95.76 JP11.12
GPIO64
  Top 0.254: U6.10 49.09,100.91 48.51,100.33 48.51,93.73 JP11.11
GPIO65
  Top 0.254: U6.17 56.51,91.07 56.9,90.68 56.9,84.33 JP11.4
GPIO66
  Top 0.254: U6.18 57.71,82.6 JP11.3
GPIO67
  Top 0.254: U7.1 80.82,111.71 JP13.20
GPIO68
  Top 0.254: U7.2 81.04,110.51 JP13.19
GPIO69
  Top 0.254: U7.4 81.82,108.11 81.53,107.82 81.53,105.92 JP13.17
GPIO70
  Top 0.254: U7.5 82.4,106.91 82.04,106.55 82.04,103.89 JP13.16
GPIO71
  Top 0.254: U7.6 82.97,105.71 82.55,105.28 82.55,101.85 JP13.15
GPIO72
  Top 0.254: U7.7 83.55,104.51 83.06,104.01 83.06,99.82 JP13.14
GPIO73
  Top 0.254: U7.8 84,103.31 83.57,102.87 83.57,97.79 JP13.13
GPIO74
  Top 0.254: U7.9 84.58,102.11 84.07,101.6 84.07,95.76 JP13.12
GPIO75
  Top 0.254: U7.10 85.16,100.91 84.58,100.33 84.58,93.73 JP13.11
GPIO76
  Top 0.254: U7.17 92.57,91.07 92.96,90.68 92.96,84.33 JP13.4
GPIO77
  Top 0.254: U7.18 93.77,82.6 JP13.3
GPIO78
  Top 0.254: U8.1 116.89,111.71 JP15.20
GPIO79
  Top 0.254: U8.2 117.11,110.51 JP15.19
GPIO80
  Top 0.254: U8.4 117.89,108.11 117.6,107.82 117.6,105.92 JP15.17
GPIO81
  Top 0.254: U8.5 118.47,106.91 118.11,106.55 118.11,103.89 JP15.16
GPIO82
  Top 0.254: U8.6 119.04,105.71 118.62,105.28 118.62,101.85 JP15.15
GPIO83
  Top 0.254: U8.7 119.62,104.51 119.13,104.01 119.13,99.82 JP15.14
GPIO84
  Top 0.254: U8.8 120.07,103.31 119.63,102.87 119.63,97.79 JP15.13
GPIO85
  Top 0.254: U8.9 120.65,102.11 120.14,101.6 120.14,95.76 JP15.12
GPIO86
  Top 0.254: U8.10 121.23,100.91 120.65,100.33 120.65,93.73 JP15.11
GPIO87
  Top 0.254: U8.17 128.64,91.07 129.03,90.68 129.03,84.33 JP15.4
GPIO88
  Top 0.254: U8.18 129.84,82.6 JP15.3
LED0  (via drill 0.51)
  Top 0.254: U1.30 32.12,43.83 37.34,38.61 37.34,34.8 38.61,33.53 JP2.10 | D1.C 17.02,29.72 v18.29,28.45
  Bottom 0.254: v18.29,28.45 28.45,28.45 30.99,30.99 38.61,30.99 JP2.10
LED1  (via drill 0.51)
  Top 0.254: U1.29 32.17,42.63 36.45,38.35 36.45,33.15 38.61,30.99 JP2.11 | D2.C 32.26,29.72 v30.99,28.45
  Bottom 0.254: v30.99,28.45 38.61,28.45 JP2.11
LED2  (via drill 0.51)
  Top 0.254: U2.30 68.19,43.83 73.41,38.61 73.41,34.8 74.68,33.53 JP4.10 | D3.C 53.09,29.72 v54.36,28.45
  Bottom 0.254: v54.36,28.45 64.52,28.45 67.06,30.99 74.68,30.99 JP4.10
LED3  (via drill 0.51)
  Top 0.254: U2.29 68.24,42.63 72.52,38.35 72.52,33.15 74.68,30.99 JP4.11 | D4.C 68.33,29.72 v67.06,28.45
  Bottom 0.254: v67.06,28.45 74.68,28.45 JP4.11
LED4  (via drill 0.51)
  Top 0.254: U3.30 104.25,43.83 109.47,38.61 109.47,34.8 110.74,33.53 JP6.10 | D5.C 89.15,29.72 v90.42,28.45
  Bottom 0.254: v90.42,28.45 100.58,28.45 103.12,30.99 110.74,30.99 JP6.10
LED5  (via drill 0.51)
  Top 0.254: U3.29 104.31,42.63 108.58,38.35 108.58,33.15 110.74,30.99 JP6.11 | D6.C 104.39,29.72 v103.12,28.45
  Bottom 0.254: v103.12,28.45 110.74,28.45 JP6.11
LED6  (via drill 0.51)
  Top 0.254: U4.30 140.32,43.83 145.54,38.61 145.54,34.8 146.81,33.53 JP8.10 | D7.C 125.22,29.72 v126.49,28.45
  Bottom 0.254: v126.49,28.45 136.65,28.45 139.19,30.99 146.81,30.99 JP8.10
LED7  (via drill 0.51)
  Top 0.254: U4.29 140.38,42.63 144.65,38.35 144.65,33.15 146.81,30.99 JP8.11 | D8.C 140.46,29.72 v139.19,28.45
  Bottom 0.254: v139.19,28.45 146.81,28.45 JP8.11
LED8  (via drill 0.51)
  Top 0.254: U5.30 32.12,99.71 37.34,94.49 37.34,90.68 38.61,89.41 JP10.10 | D9.C 17.02,85.6 v18.29,84.33
  Bottom 0.254: v18.29,84.33 28.45,84.33 30.99,86.87 38.61,86.87 JP10.10
LED9  (via drill 0.51)
  Top 0.254: U5.29 32.17,98.51 36.45,94.23 36.45,89.03 38.61,86.87 JP10.11 | D10.C 32.26,85.6 v30.99,84.33
  Bottom 0.254: v30.99,84.33 38.61,84.33 JP10.11
LED10  (via drill 0.51)
  Top 0.254: U6.30 68.19,99.71 73.41,94.49 73.41,90.68 74.68,89.41 JP12.10 | D11.C 53.09,85.6 v54.36,84.33
  Bottom 0.254: v54.36,84.33 64.52,84.33 67.06,86.87 74.68,86.87 JP12.10
LED11  (via drill 0.51)
  Top 0.254: U6.29 68.24,98.51 72.52,94.23 72.52,89.03 74.68,86.87 JP12.11 | D12.C 68.33,85.6 v67.06,84.33
  Bottom 0.254: v67.06,84.33 74.68,84.33 JP12.11
LED12  (via drill 0.51)
  Top 0.254: U7.30 104.25,99.71 109.47,94.49 109.47,90.68 110.74,89.41 JP14.10 | D13.C 89.15,85.6 v90.42,84.33
  Bottom 0.254: v90.42,84.33 100.58,84.33 103.12,86.87 110.74,86.87 JP14.10
LED13  (via drill 0.51)
  Top 0.254: U7.29 104.31,98.51 108.58,94.23 108.58,89.03 110.74,86.87 JP14.11 | D14.C 104.39,85.6 v103.12,84.33
  Bottom 0.254: v103.12,84.33 110.74,84.33 JP14.11
LED14  (via drill 0.51)
  Top 0.254: U8.30 140.32,99.71 145.54,94.49 145.54,90.68 146.81,89.41 JP16.10 | D15.C 125.22,85.6 v126.49,84.33
  Bottom 0.254: v126.49,84.33 136.65,84.33 139.19,86.87 146.81,86.87 JP16.10
LED15  (via drill 0.51)
  Top 0.254: U8.29 140.38,98.51 144.65,94.23 144.65,89.03 146.81,86.87 JP16.11 | D16.C 140.46,85.6 v139.19,84.33
  Bottom 0.254: v139.19,84.33 146.81,84.33 JP16.11
MIC_BIAS
  Top 0.254: U1.31 33.46,45.03 38.61,39.88 38.61,37.34 39.88,36.07 JP2.9
MIC_BIAS1
  Top 0.254: U2.31 69.53,45.03 74.68,39.88 74.68,37.34 75.95,36.07 JP4.9
MIC_BIAS2
  Top 0.254: U3.31 105.59,45.03 110.74,39.88 110.74,37.34 112.01,36.07 JP6.9
MIC_BIAS3
  Top 0.254: U4.31 141.66,45.03 146.81,39.88 146.81,37.34 148.08,36.07 JP8.9
MIC_BIAS4
  Top 0.254: U5.31 33.46,100.91 38.61,95.76 38.61,93.22 39.88,91.95 JP10.9
MIC_BIAS5
  Top 0.254: U6.31 69.53,100.91 74.68,95.76 74.68,93.22 75.95,91.95 JP12.9
MIC_BIAS6
  Top 0.254: U7.31 105.59,100.91 110.74,95.76 110.74,93.22 112.01,91.95 JP14.9
MIC_BIAS7
  Top 0.254: U8.31 141.66,100.91 146.81,95.76 146.81,93.22 148.08,91.95 JP16.9
MIC_L+
  Top 0.254: U1.32 35.31,46.23 39.88,41.66 39.88,39.88 JP2.8
MIC_L+1
  Top 0.254: U2.32 71.37,46.23 75.95,41.66 75.95,39.88 JP4.8
MIC_L+2
  Top 0.254: U3.32 107.44,46.23 112.01,41.66 112.01,39.88 JP6.8
MIC_L+3
  Top 0.254: U4.32 143.51,46.23 148.08,41.66 148.08,39.88 JP8.8
MIC_L+4
  Top 0.254: U5.32 35.31,102.11 39.88,97.54 39.88,95.76 JP10.8
MIC_L+5
  Top 0.254: U6.32 71.37,102.11 75.95,97.54 75.95,95.76 JP12.8
MIC_L+6
  Top 0.254: U7.32 107.44,102.11 112.01,97.54 112.01,95.76 JP14.8
MIC_L+7
  Top 0.254: U8.32 143.51,102.11 148.08,97.54 148.08,95.76 JP16.8
MIC_L-
  Top 0.254: U1.34 36.84,48.63 40.51,44.96 40.51,44.32 JP2.6
MIC_L-1
  Top 0.254: U2.34 72.91,48.63 76.58,44.96 76.58,44.32 JP4.6
MIC_L-2
  Top 0.254: U3.34 108.98,48.63 112.65,44.96 112.65,44.32 JP6.6
MIC_L-3
  Top 0.254: U4.34 145.05,48.63 148.72,44.96 148.72,44.32 JP8.6
MIC_L-4
  Top 0.254: U5.34 36.84,104.51 40.51,100.84 40.51,100.2 JP10.6
MIC_L-5
  Top 0.254: U6.34 72.91,104.51 76.58,100.84 76.58,100.2 JP12.6
MIC_L-6
  Top 0.254: U7.34 108.98,104.51 112.65,100.84 112.65,100.2 JP14.6
MIC_L-7
  Top 0.254: U8.34 145.05,104.51 148.72,100.84 148.72,100.2 JP16.6
MIC_R+
  Top 0.254: U1.33 36.65,47.43 39.88,44.2 39.88,42.42 JP2.7
MIC_R+1
  Top 0.254: U2.33 72.71,47.43 75.95,44.2 75.95,42.42 JP4.7
MIC_R+2
  Top 0.254: U3.33 108.78,47.43 112.01,44.2 112.01,42.42 JP6.7
MIC_R+3
  Top 0.254: U4.33 144.85,47.43 148.08,44.2 148.08,42.42 JP8.7
MIC_R+4
  Top 0.254: U5.33 36.65,103.31 39.88,100.08 39.88,98.3 JP10.7
MIC_R+5
  Top 0.254: U6.33 72.71,103.31 75.95,100.08 75.95,98.3 JP12.7
MIC_R+6
  Top 0.254: U7.33 108.78,103.31 112.01,100.08 112.01,98.3 JP14.7
MIC_R+7
  Top 0.254: U8.33 144.85,103.31 148.08,100.08 148.08,98.3 JP16.7
MIC_R-
  Top 0.254: U1.35 31.2,49.83 30.99,50.04 37.97,50.04 40.51,47.5 40.51,46.86 JP2.5
MIC_R-1
  Top 0.254: U2.35 67.27,49.83 67.06,50.04 74.04,50.04 76.58,47.5 76.58,46.86 JP4.5
MIC_R-2
  Top 0.254: U3.35 103.33,49.83 103.12,50.04 110.11,50.04 112.65,47.5 112.65,46.86 JP6.5
MIC_R-3
  Top 0.254: U4.35 139.4,49.83 139.19,50.04 146.18,50.04 148.72,47.5 148.72,46.86 JP8.5
MIC_R-4
  Top 0.254: U5.35 31.2,105.71 30.99,105.92 37.97,105.92 40.51,103.38 40.51,102.74 JP10.5
MIC_R-5
  Top 0.254: U6.35 67.27,105.71 67.06,105.92 74.04,105.92 76.58,103.38 76.58,102.74 JP12.5
MIC_R-6
  Top 0.254: U7.35 103.33,105.71 103.12,105.92 110.11,105.92 112.65,103.38 112.65,102.74 JP14.5
MIC_R-7
  Top 0.254: U8.35 139.4,105.71 139.19,105.92 146.18,105.92 148.72,103.38 148.72,102.74 JP16.5
N$1
  Top 0.254: D2.A 31.74,31.74 30.14,30.14 R2.1
N$2
  Top 0.254: D1.A 17.54,31.74 19.14,30.14 R1.1
N$3
  Top 0.254: D4.A 67.81,31.74 66.21,30.14 R4.1
N$4
  Top 0.254: D3.A 53.61,31.74 55.21,30.14 R3.1
N$5
  Top 0.254: D6.A 103.87,31.74 102.27,30.14 R6.1
N$6
  Top 0.254: D5.A 89.67,31.74 91.27,30.14 R5.1
N$7
  Top 0.254: D8.A 139.94,31.74 138.34,30.14 R8.1
N$8
  Top 0.254: D7.A 125.74,31.74 127.34,30.14 R7.1
N$9
  Top 0.254: D10.A 31.74,87.62 30.14,86.02 R10.1
N$10
  Top 0.254: D9.A 17.54,87.62 19.14,86.02 R9.1
N$11
  Top 0.254: D12.A 67.81,87.62 66.21,86.02 R12.1
N$12
  Top 0.254: D11.A 53.61,87.62 55.21,86.02 R11.1
N$13
  Top 0.254: D14.A 103.87,87.62 102.27,86.02 R14.1
N$14
  Top 0.254: D13.A 89.67,87.62 91.27,86.02 R13.1
N$15
  Top 0.254: D16.A 139.94,87.62 138.34,86.02 R16.1
N$16
  Top 0.254: D15.A 125.74,87.62 127.34,86.02 R15.1
PCM_CLK
  Top 0.254: JP2.16 38.61,18.29 28.45,28.45 28.45,34.8 28.84,35.19 U1.24
PCM_CLK1
  Top 0.254: JP4.16 74.68,18.29 64.52,28.45 64.52,34.8 64.91,35.19 U2.24
PCM_CLK2
  Top 0.254: JP6.16 110.74,18.29 100.58,28.45 100.58,34.8 100.97,35.19 U3.24
PCM_CLK3
  Top 0.254: JP8.16 146.81,18.29 136.65,28.45 136.65,34.8 137.04,35.19 U4.24
PCM_CLK4
  Top 0.254: JP10.16 38.61,74.17 28.45,84.33 28.45,90.68 28.84,91.07 U5.24
PCM_CLK5
  Top 0.254: JP12.16 74.68,74.17 64.52,84.33 64.52,90.68 64.91,91.07 U6.24
PCM_CLK6
  Top 0.254: JP14.16 110.74,74.17 100.58,84.33 100.58,90.68 100.97,91.07 U7.24
PCM_CLK7
  Top 0.254: JP16.16 146.81,74.17 136.65,84.33 136.65,90.68 137.04,91.07 U8.24
PCM_IN
  Top 0.254: U1.21 25.24,24.04 38.61,10.67 JP2.19
PCM_IN1
  Top 0.254: U2.21 61.31,24.04 74.68,10.67 JP4.19
PCM_IN2
  Top 0.254: U3.21 97.37,24.04 110.74,10.67 JP6.19
PCM_IN3
  Top 0.254: U4.21 133.44,24.04 146.81,10.67 JP8.19
PCM_IN4
  Top 0.254: U5.21 25.24,79.92 38.61,66.55 JP10.19
PCM_IN5
  Top 0.254: U6.21 61.31,79.92 74.68,66.55 JP12.19
PCM_IN6
  Top 0.254: U7.21 97.37,79.92 110.74,66.55 JP14.19
PCM_IN7
  Top 0.254: U8.21 133.44,79.92 146.81,66.55 JP16.19
PCM_OUT
  Top 0.254: U1.22 26.44,25.38 38.61,13.21 JP2.18
PCM_OUT1
  Top 0.254: U2.22 62.51,25.38 74.68,13.21 JP4.18
PCM_OUT2
  Top 0.254: U3.22 98.57,25.38 110.74,13.21 JP6.18
PCM_OUT3
  Top 0.254: U4.22 134.64,25.38 146.81,13.21 JP8.18
PCM_OUT4
  Top 0.254: U5.22 26.44,81.26 38.61,69.09 JP10.18
PCM_OUT5
  Top 0.254: U6.22 62.51,81.26 74.68,69.09 JP12.18
PCM_OUT6
  Top 0.254: U7.22 98.57,81.26 110.74,69.09 JP14.18
PCM_OUT7
  Top 0.254: U8.22 134.64,81.26 146.81,69.09 JP16.18
PCM_SYNC
  Top 0.254: U1.23 27.64,26.72 38.61,15.75 JP2.17
PCM_SYNC1
  Top 0.254: U2.23 63.71,26.72 74.68,15.75 JP4.17
PCM_SYNC2
  Top 0.254: U3.23 99.77,26.72 110.74,15.75 JP6.17
PCM_SYNC3
  Top 0.254: U4.23 135.84,26.72 146.81,15.75 JP8.17
PCM_SYNC4
  Top 0.254: U5.23 27.64,82.6 38.61,71.63 JP10.17
PCM_SYNC5
  Top 0.254: U6.23 63.71,82.6 74.68,71.63 JP12.17
PCM_SYNC6
  Top 0.254: U7.23 99.77,82.6 110.74,71.63 JP14.17
PCM_SYNC7
  Top 0.254: U8.23 135.84,82.6 146.81,71.63 JP16.17
PWREN
  Top 0.254: U1.19 22.84,25.38 JP1.2
PWREN1
  Top 0.254: U2.19 58.91,25.38 JP3.2
PWREN2
  Top 0.254: U3.19 94.97,25.38 JP5.2
PWREN3
  Top 0.254: U4.19 131.04,25.38 JP7.2
PWREN4
  Top 0.254: U5.19 22.84,81.26 JP9.2
PWREN5
  Top 0.254: U6.19 58.91,81.26 JP11.2
PWREN6
  Top 0.254: U7.19 94.97,81.26 JP13.2
PWREN7
  Top 0.254: U8.19 131.04,81.26 JP15.2
SPI_CLK
  Top 0.254: U1.27 32.42,40.23 35.05,37.59 35.05,30.73 39.88,25.91 JP2.13
SPI_CLK1
  Top 0.254: U2.27 68.48,40.23 71.12,37.59 71.12,30.73 75.95,25.91 JP4.13
SPI_CLK2
  Top 0.254: U3.27 104.55,40.23 107.19,37.59 107.19,30.73 112.01,25.91 JP6.13
SPI_CLK3
  Top 0.254: U4.27 140.62,40.23 143.26,37.59 143.26,30.73 148.08,25.91 JP8.13
SPI_CLK4
  Top 0.254: U5.27 32.42,96.11 35.05,93.47 35.05,86.61 39.88,81.79 JP10.13
SPI_CLK5
  Top 0.254: U6.27 68.48,96.11 71.12,93.47 71.12,86.61 75.95,81.79 JP12.13
SPI_CLK6
  Top 0.254: U7.27 104.55,96.11 107.19,93.47 107.19,86.61 112.01,81.79 JP14.13
SPI_CLK7
  Top 0.254: U8.27 140.62,96.11 143.26,93.47 143.26,86.61 148.08,81.79 JP16.13
SPI_MISO
  Top 0.254: U1.26 32.73,39.03 34.29,37.47 34.29,28.96 39.88,23.37 JP2.14
SPI_MISO1
  Top 0.254: U2.26 68.8,39.03 70.36,37.47 70.36,28.96 75.95,23.37 JP4.14
SPI_MISO2
  Top 0.254: U3.26 104.86,39.03 106.43,37.47 106.43,28.96 112.01,23.37 JP6.14
SPI_MISO3
  Top 0.254: U4.26 140.93,39.03 142.49,37.47 142.49,28.96 148.08,23.37 JP8.14
SPI_MISO4
  Top 0.254: U5.26 32.73,94.91 34.29,93.34 34.29,84.84 39.88,79.25 JP10.14
SPI_MISO5
  Top 0.254: U6.26 68.8,94.91 70.36,93.34 70.36,84.84 75.95,79.25 JP12.14
SPI_MISO6
  Top 0.254: U7.26 104.86,94.91 106.43,93.34 106.43,84.84 112.01,79.25 JP14.14
SPI_MISO7
  Top 0.254: U8.26 140.93,94.91 142.49,93.34 142.49,84.84 148.08,79.25 JP16.14
SPI_MOSI
  Top 0.254: U1.28 32.23,41.43 35.69,37.97 35.69,31.37 38.61,28.45 JP2.12
SPI_MOSI1
  Top 0.254: U2.28 68.3,41.43 71.75,37.97 71.75,31.37 74.68,28.45 JP4.12
SPI_MOSI2
  Top 0.254: U3.28 104.37,41.43 107.82,37.97 107.82,31.37 110.74,28.45 JP6.12
SPI_MOSI3
  Top 0.254: U4.28 140.44,41.43 143.89,37.97 143.89,31.37 146.81,28.45 JP8.12
SPI_MOSI4
  Top 0.254: U5.28 32.23,97.31 35.69,93.85 35.69,87.25 38.61,84.33 JP10.12
SPI_MOSI5
  Top 0.254: U6.28 68.3,97.31 71.75,93.85 71.75,87.25 74.68,84.33 JP12.12
SPI_MOSI6
  Top 0.254: U7.28 104.37,97.31 107.82,93.85 107.82,87.25 110.74,84.33 JP14.12
SPI_MOSI7
  Top 0.254: U8.28 140.44,97.31 143.89,93.85 143.89,87.25 146.81,84.33 JP16.12
SPI_SS
  Top 0.254: U1.25 33.04,37.83 33.53,37.34 33.53,27.18 39.88,20.83 JP2.15
SPI_SS1
  Top 0.254: U2.25 69.11,37.83 69.6,37.34 69.6,27.18 75.95,20.83 JP4.15
SPI_SS2
  Top 0.254: U3.25 105.17,37.83 105.66,37.34 105.66,27.18 112.01,20.83 JP6.15
SPI_SS3
  Top 0.254: U4.25 141.24,37.83 141.73,37.34 141.73,27.18 148.08,20.83 JP8.15
SPI_SS4
  Top 0.254: U5.25 33.04,93.71 33.53,93.22 33.53,83.06 39.88,76.71 JP10.15
SPI_SS5
  Top 0.254: U6.25 69.11,93.71 69.6,93.22 69.6,83.06 75.95,76.71 JP12.15
SPI_SS6
  Top 0.254: U7.25 105.17,93.71 105.66,93.22 105.66,83.06 112.01,76.71 JP14.15
SPI_SS7
  Top 0.254: U8.25 141.24,93.71 141.73,93.22 141.73,83.06 148.08,76.71 JP16.15
SPKR_L+
  Top 0.254: U1.40 40.59,55.83 JP2.1
SPKR_L+1
  Top 0.254: U2.40 76.66,55.83 JP4.1
SPKR_L+2
  Top 0.254: U3.40 112.72,55.83 JP6.1
SPKR_L+3
  Top 0.254: U4.40 148.79,55.83 JP8.1
SPKR_L+4
  Top 0.254: U5.40 40.59,111.71 JP10.1
SPKR_L+5
  Top 0.254: U6.40 76.66,111.71 JP12.1
SPKR_L+6
  Top 0.254: U7.40 112.72,111.71 JP14.1
SPKR_L+7
  Top 0.254: U8.40 148.79,111.71 JP16.1
SPKR_L-
  Top 0.254: U1.38 39.66,53.43 41.15,51.94 JP2.3
SPKR_L-1
  Top 0.254: U2.38 75.73,53.43 77.22,51.94 JP4.3
SPKR_L-2
  Top 0.254: U3.38 111.8,53.43 113.28,51.94 JP6.3
SPKR_L-3
  Top 0.254: U4.38 147.87,53.43 149.35,51.94 JP8.3
SPKR_L-4
  Top 0.254: U5.38 39.66,109.31 41.15,107.82 JP10.3
SPKR_L-5
  Top 0.254: U6.38 75.73,109.31 77.22,107.82 JP12.3
SPKR_L-6
  Top 0.254: U7.38 111.8,109.31 113.28,107.82 JP14.3
SPKR_L-7
  Top 0.254: U8.38 147.87,109.31 149.35,107.82 JP16.3
SPKR_R+
  Top 0.254: U1.39 40.37,54.63 JP2.2
SPKR_R+1
  Top 0.254: U2.39 76.44,54.63 JP4.2
SPKR_R+2
  Top 0.254: U3.39 112.5,54.63 JP6.2
SPKR_R+3
  Top 0.254: U4.39 148.57,54.63 JP8.2
SPKR_R+4
  Top 0.254: U5.39 40.37,110.51 JP10.2
SPKR_R+5
  Top 0.254: U6.39 76.44,110.51 JP12.2
SPKR_R+6
  Top 0.254: U7.39 112.5,110.51 JP14.2
SPKR_R+7
  Top 0.254: U8.39 148.57,110.51 JP16.2
SPKR_R-
  Top 0.254: U1.37 38.96,52.23 39.88,51.31 39.88,50.04 JP2.4
SPKR_R-1
  Top 0.254: U2.37 75.03,52.23 75.95,51.31 75.95,50.04 JP4.4
SPKR_R-2
  Top 0.254: U3.37 111.09,52.23 112.01,51.31 112.01,50.04 JP6.4
SPKR_R-3
  Top 0.254: U4.37 147.16,52.23 148.08,51.31 148.08,50.04 JP8.4
SPKR_R-4
  Top 0.254: U5.37 38.96,108.11 39.88,107.19 39.88,105.92 JP10.4
SPKR_R-5
  Top 0.254: U6.37 75.03,108.11 75.95,107.19 75.95,105.92 JP12.4
SPKR_R-6
  Top 0.254: U7.37 111.09,108.11 112.01,107.19 112.01,105.92 JP14.4
SPKR_R-7
  Top 0.254: U8.37 147.16,108.11 148.08,107.19 148.08,105.92 JP16.4
UART_CTS
  Top 0.254: U1.14 15.34,40.23 14.48,39.37 14.48,29.72 JP1.7
UART_CTS1
  Top 0.254: U2.14 51.4,40.23 50.55,39.37 50.55,29.72 JP3.7
UART_CTS2
  Top 0.254: U3.14 87.47,40.23 86.61,39.37 86.61,29.72 JP5.7
UART_CTS3
  Top 0.254: U4.14 123.54,40.23 122.68,39.37 122.68,29.72 JP7.7
UART_CTS4
  Top 0.254: U5.14 15.34,96.11 14.48,95.25 14.48,85.6 JP9.7
UART_CTS5
  Top 0.254: U6.14 51.4,96.11 50.55,95.25 50.55,85.6 JP11.7
UART_CTS6
  Top 0.254: U7.14 87.47,96.11 86.61,95.25 86.61,85.6 JP13.7
UART_CTS7
  Top 0.254: U8.14 123.54,96.11 122.68,95.25 122.68,85.6 JP15.7
UART_RTS
  Top 0.254: U1.13 15.52,41.43 13.97,39.88 13.97,31.75 JP1.8
UART_RTS1
  Top 0.254: U2.13 51.59,41.43 50.04,39.88 50.04,31.75 JP3.8
UART_RTS2
  Top 0.254: U3.13 87.66,41.43 86.11,39.88 86.11,31.75 JP5.8
UART_RTS3
  Top 0.254: U4.13 123.72,41.43 122.17,39.88 122.17,31.75 JP7.8
UART_RTS4
  Top 0.254: U5.13 15.52,97.31 13.97,95.76 13.97,87.63 JP9.8
UART_RTS5
  Top 0.254: U6.13 51.59,97.31 50.04,95.76 50.04,87.63 JP11.8
UART_RTS6
  Top 0.254: U7.13 87.66,97.31 86.11,95.76 86.11,87.63 JP13.8
UART_RTS7
  Top 0.254: U8.13 123.72,97.31 122.17,95.76 122.17,87.63 JP15.8
UART_RX
  Top 0.254: U1.16 16.24,37.83 15.75,37.34 15.75,25.91 JP1.5
UART_RX1
  Top 0.254: U2.16 52.31,37.83 51.82,37.34 51.82,25.91 JP3.5
UART_RX2
  Top 0.254: U3.16 88.37,37.83 87.88,37.34 87.88,25.91 JP5.5
UART_RX3
  Top 0.254: U4.16 124.44,37.83 123.95,37.34 123.95,25.91 JP7.5
UART_RX4
  Top 0.254: U5.16 16.24,93.71 15.75,93.22 15.75,81.79 JP9.5
UART_RX5
  Top 0.254: U6.16 52.31,93.71 51.82,93.22 51.82,81.79 JP11.5
UART_RX6
  Top 0.254: U7.16 88.37,93.71 87.88,93.22 87.88,81.79 JP13.5
UART_RX7
  Top 0.254: U8.16 124.44,93.71 123.95,93.22 123.95,81.79 JP15.5
UART_TX
  Top 0.254: U1.15 15.53,39.03 14.99,38.48 14.99,27.69 JP1.6
UART_TX1
  Top 0.254: U2.15 51.6,39.03 51.05,38.48 51.05,27.69 JP3.6
UART_TX2
  Top 0.254: U3.15 87.67,39.03 87.12,38.48 87.12,27.69 JP5.6
UART_TX3
  Top 0.254: U4.15 123.74,39.03 123.19,38.48 123.19,27.69 JP7.6
UART_TX4
  Top 0.254: U5.15 15.53,94.91 14.99,94.36 14.99,83.57 JP9.6
UART_TX5
  Top 0.254: U6.15 51.6,94.91 51.05,94.36 51.05,83.57 JP11.6
UART_TX6
  Top 0.254: U7.15 87.67,94.91 87.12,94.36 87.12,83.57 JP13.6
UART_TX7
  Top 0.254: U8.15 123.74,94.91 123.19,94.36 123.19,83.57 JP15.6
USBD+
  Top 0.254: U1.12 13.93,42.63 13.46,42.16 13.46,33.78 JP1.9
USBD+1
  Top 0.254: U2.12 49.99,42.63 49.53,42.16 49.53,33.78 JP3.9
USBD+2
  Top 0.254: U3.12 86.06,42.63 85.6,42.16 85.6,33.78 JP5.9
USBD+3
  Top 0.254: U4.12 122.13,42.63 121.67,42.16 121.67,33.78 JP7.9
USBD+4
  Top 0.254: U5.12 13.93,98.51 13.46,98.04 13.46,89.66 JP9.9
USBD+5
  Top 0.254: U6.12 49.99,98.51 49.53,98.04 49.53,89.66 JP11.9
USBD+6
  Top 0.254: U7.12 86.06,98.51 85.6,98.04 85.6,89.66 JP13.9
USBD+7
  Top 0.254: U8.12 122.13,98.51 121.67,98.04 121.67,89.66 JP15.9
USBD-
  Top 0.254: U1.11 13.6,43.83 12.95,43.18 12.95,35.81 JP1.10
USBD-1
  Top 0.254: U2.11 49.67,43.83 49.02,43.18 49.02,35.81 JP3.10
USBD-2
  Top 0.254: U3.11 85.74,43.83 85.09,43.18 85.09,35.81 JP5.10
USBD-3
  Top 0.254: U4.11 121.81,43.83 121.16,43.18 121.16,35.81 JP7.10
USBD-4
  Top 0.254: U5.11 13.6,99.71 12.95,99.06 12.95,91.69 JP9.10
USBD-5
  Top 0.254: U6.11 49.67,99.71 49.02,99.06 49.02,91.69 JP11.10
USBD-6
  Top 0.254: U7.11 85.74,99.71 85.09,99.06 85.09,91.69 JP13.10
USBD-7
  Top 0.254: U8.11 121.81,99.71 121.16,99.06 121.16,91.69 JP15.10

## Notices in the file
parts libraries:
SparkFun-RF: Licensing: CC v3.0 Share-Alike You are welcome to use this library for commercial purposes.
